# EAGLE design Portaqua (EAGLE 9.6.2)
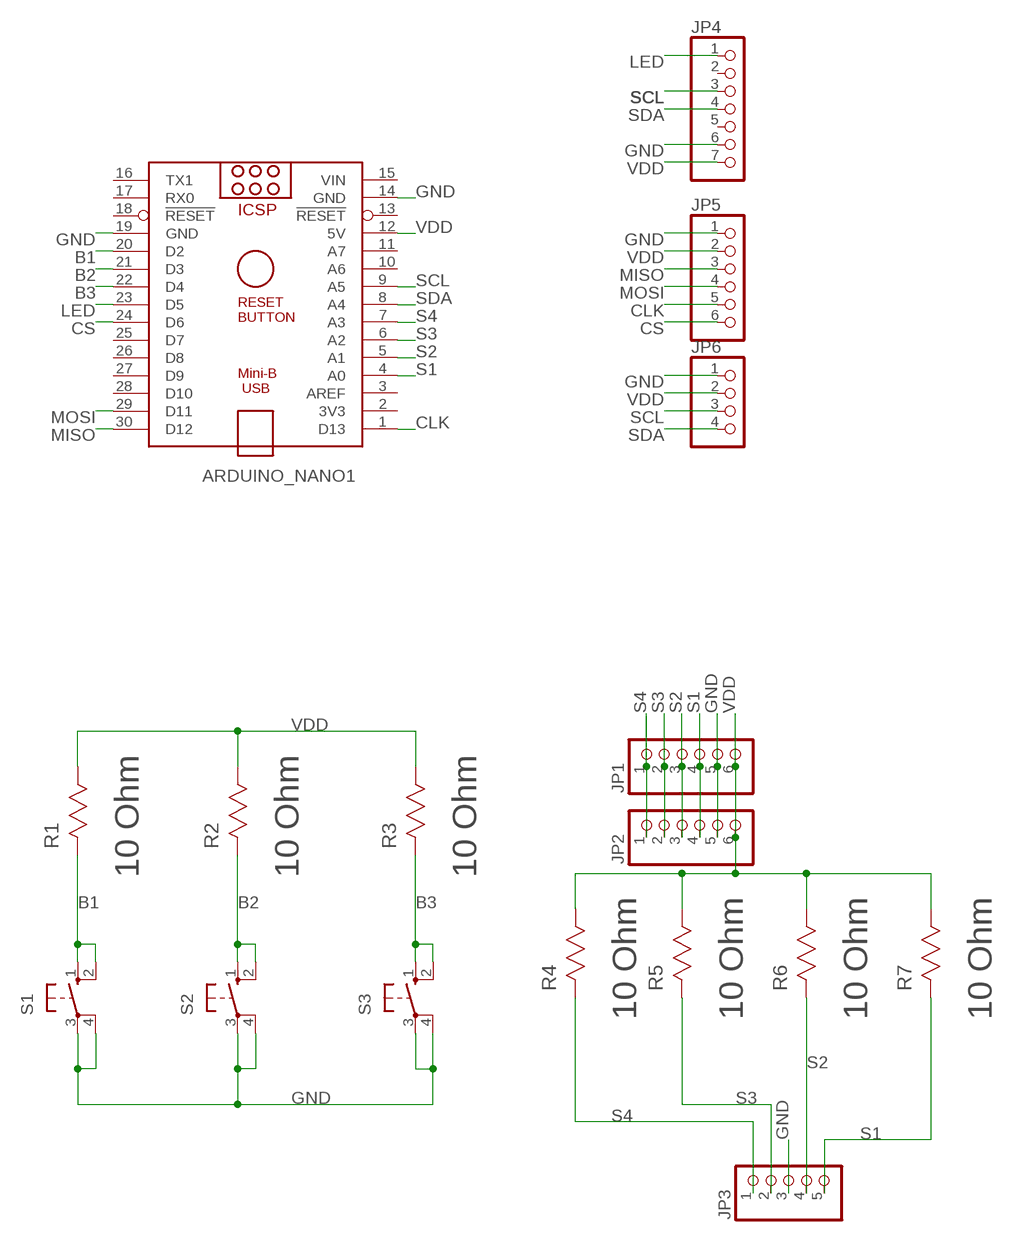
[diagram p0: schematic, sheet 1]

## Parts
ARDUINO_NANO1  ARDUINO_NANO  [ARDUINO_NANO]
JP1  PINHD-1X6  [1X06]
JP2  PINHD-1X6  [1X06]
JP3  PINHD-1X05_2.54-SMD-90°  [1X05SMD/90]
JP4  PINHD-1X7  [1X07]
JP5  PINHD-1X6  [1X06]
JP6  PINHD-1X4  [1X04]
R1  10 Ohm  CRM1206-FX-10R0ELF  [RESC3216X71N]
R2  10 Ohm  CRM1206-FX-10R0ELF  [RESC3216X71N]
R3  10 Ohm  CRM1206-FX-10R0ELF  [RESC3216X71N]
R4  10 Ohm  CRM1206-FX-10R0ELF  [RESC3216X71N]
R5  10 Ohm  CRM1206-FX-10R0ELF  [RESC3216X71N]
R6  10 Ohm  CRM1206-FX-10R0ELF  [RESC3216X71N]
R7  10 Ohm  CRM1206-FX-10R0ELF  [RESC3216X71N]
S1  10-XX  [B3F-10XX]
S2  10-XX  [B3F-10XX]
S3  10-XX  [B3F-10XX]

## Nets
B1: ARDUINO_NANO1.20(D2) R1.2(R2) S1.1(S) S1.2(S1)
B2: ARDUINO_NANO1.21(D3) R2.2(R2) S2.1(S) S2.2(S1)
B3: ARDUINO_NANO1.22(D4) R3.2(R2) S3.1(S) S3.2(S1)
CLK: ARDUINO_NANO1.1(D13) JP5.5
CS: ARDUINO_NANO1.24(D6) JP5.6
GND: ARDUINO_NANO1.14(GND) ARDUINO_NANO1.19(GND) JP1.5 JP2.5 JP3.3 JP4.6 JP5.1 JP6.1 S1.3(P) S1.4(P1) S2.3(P) S2.4(P1) S3.3(P) S3.4(P1)
LED: ARDUINO_NANO1.23(D5) JP4.1
MISO: ARDUINO_NANO1.30(D12) JP5.3
MOSI: ARDUINO_NANO1.29(D11) JP5.4
S1: ARDUINO_NANO1.4(A0) JP1.4 JP2.4 JP3.5 R7.2(R2)
S2: ARDUINO_NANO1.5(A1) JP1.3 JP2.3 JP3.4 R6.2(R2)
S3: ARDUINO_NANO1.6(A2) JP1.2 JP2.2 JP3.2 R5.2(R2)
S4: ARDUINO_NANO1.7(A3) JP1.1 JP2.1 JP3.1 R4.2(R2)
SCL: ARDUINO_NANO1.9(A5) JP4.3 JP6.3
SDA: ARDUINO_NANO1.8(A4) JP4.4 JP6.4
VDD: ARDUINO_NANO1.12(5V) JP1.6 JP2.6 JP4.7 JP5.2 JP6.2 R1.1(R1) R2.1(R1) R3.1(R1) R4.1(R1) R5.1(R1) R6.1(R1) R7.1(R1)
Unconnected: ARDUINO_NANO1.2(3V3) ARDUINO_NANO1.3(AREF) ARDUINO_NANO1.10(A6) ARDUINO_NANO1.11(A7) ARDUINO_NANO1.13(!RESET) ARDUINO_NANO1.16(TX1) ARDUINO_NANO1.17(RX0) ARDUINO_NANO1.18(!RESET) ARDUINO_NANO1.25(D7) ARDUINO_NANO1.26(D8) ARDUINO_NANO1.27(D9) ARDUINO_NANO1.28(D10) JP4.2 JP4.5

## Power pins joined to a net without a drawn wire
VIN: ARDUINO_NANO1.15(VIN)

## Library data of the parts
ARDUINO_NANO1 = ArduinoNanoV30:ARDUINO_NANO: Arduino Nano V3.0 Overview: The Arduino Nano is a small, complete, and breadboard-friendly board based on the ATmega328 (Arduino Nano 3.x) or ATmega168 (Arduino Nano 2.x). It has more or less the same functionality of the Arduino Duemilanove, but in a different package. It lacks only a DC power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
JP1 JP2 JP5 = pinhead:PINHD-1X6: PIN HEADER
JP3 = pinhead-2:PINHD-1X05: PIN HEADER
JP4 = pinhead:PINHD-1X7: PIN HEADER
JP6 = pinhead:PINHD-1X4: PIN HEADER
R1-R7 = Bourns_By_element14_Batch_1:CRM1206-FX-10R0ELF: Resistor 1206; MPN: CRM1206-FX-10R0ELF; OC_FARNELL: 1865248; OC_NEWARK: 17T4257; SUPPLIER: BOURNS; TOLERANCE: ±1 %; WATTAGE: 0.5W
S1-S3 = switch-omron:10-XX: OMRON SWITCH; MPN: B3F-1000; OC_FARNELL: 176432; OC_NEWARK: 36M3542

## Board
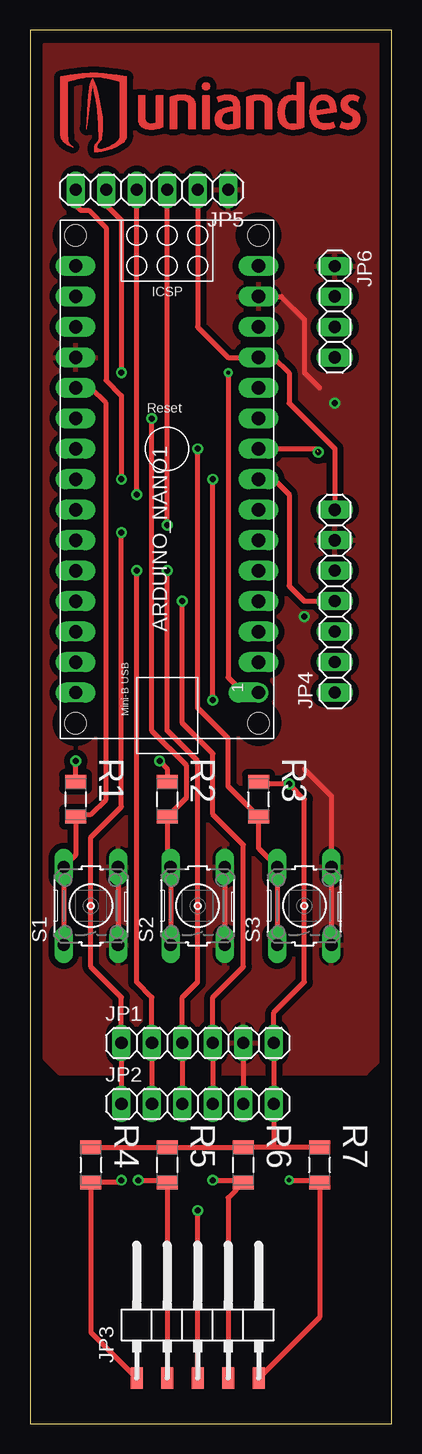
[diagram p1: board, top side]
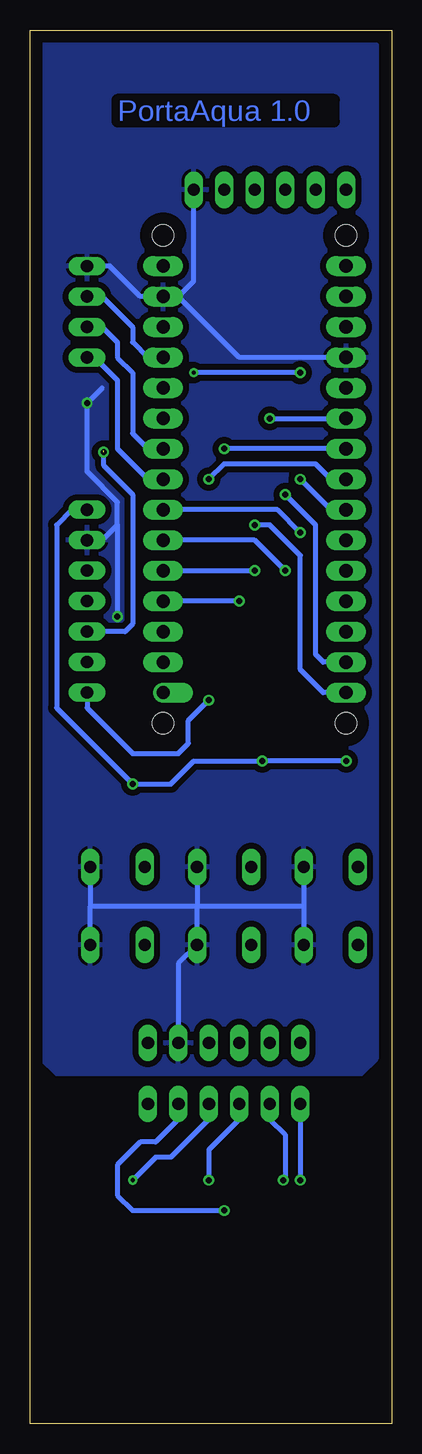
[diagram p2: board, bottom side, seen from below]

Size 30.15 x 116.2 mm. Coordinates in mm from the lower left corner, seen from the top.
Outline: 0,0 30.15,0 30.15,116.2 0,116.2 0,0
Copper layers (1*16): Top 0.035mm / dielectric 1.5mm / Bottom 0.035mm
Design rules "default *": minimum track width 6mil, minimum drill 0.35mm, track to track 20mil, track to pad 20mil, pad to pad 20mil, via to via 20mil, smd to smd 20mil, copper to edge 40mil, drill to drill 6mil, minimum pad ring 10mil, minimum via ring 8mil, stop-mask expansion 4mil, vias tented up to drill 0mil, thermal gap 10mil

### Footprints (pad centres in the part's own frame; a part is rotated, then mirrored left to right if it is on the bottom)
ARDUINO_NANO = drill 1.11 offset: 1 -20.32,-7.62 | drill 1.11 long: 2 -17.78,-7.62; 3 -15.24,-7.62; 4 -12.7,-7.62; 5 -10.16,-7.62; 6 -7.62,-7.62; 7 -5.08,-7.62; 8 -2.54,-7.62; 9 0,-7.62; 10 2.54,-7.62; 11 5.08,-7.62; 12 7.62,-7.62; 13 10.16,-7.62; 14 12.7,-7.62; 15 15.24,-7.62; 16 15.24,7.62; 17 12.7,7.62; 18 10.16,7.62; 19 7.62,7.62; 20 5.08,7.62; 21 2.54,7.62; 22 0,7.62; 23 -2.54,7.62; 24 -5.08,7.62; 25 -7.62,7.62; 26 -10.16,7.62; 27 -12.7,7.62; 28 -15.24,7.62; 29 -17.78,7.62; 30 -20.32,7.62 | hole 1.778: -22.86,-7.62; -22.86,7.62; 17.78,7.62; 17.78,-7.62
1X06 = drill 1.016 long: 1 -6.35,0; 2 -3.81,0; 3 -1.27,0; 4 1.27,0; 5 3.81,0; 6 6.35,0
1X05SMD/90 = smd 1.016 x 1.778: 1 -1.27,-5.08; 2 1.27,-5.08; 3 3.81,-5.08; 4 6.35,-5.08; 5 8.89,-5.08
1X07 = drill 1.016 long: 1 -7.62,0; 2 -5.08,0; 3 -2.54,0; 4 0,0; 5 2.54,0; 6 5.08,0; 7 7.62,0
1X04 = drill 1.016 long: 1 -3.81,0; 2 -1.27,0; 3 1.27,0; 4 3.81,0
RESC3216X71N = smd 1.118 x 1.753: 1 -1.473,0; 2 1.473,0
B3F-10XX = drill 1.016 long: 1 -3.251,2.261; 2 3.251,2.261; 3 -3.251,-2.261; 4 3.251,-2.261

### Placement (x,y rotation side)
ARDUINO_NANO1  11.43,81.28 90 top
JP1  13.97,31.75 0 top
JP2  13.97,26.67 0 top
JP3  10.16,8.89 0 top
JP4  25.4,68.58 90 top
JP5  10.16,102.87 180 top
JP6  25.4,92.71 270 top
R1  3.81,52.07 270 top
R2  11.43,52.07 270 top
R3  19.05,52.07 270 top
R4  5.08,21.59 270 top
R5  11.43,21.59 270 top
R6  17.78,21.59 270 top
R7  24.13,21.59 270 top
S1  5.08,43.18 90 top
S2  13.97,43.18 90 top
S3  22.86,43.18 90 top
U$1  [UNIANDES25MM]  2.54,106.05 0 top

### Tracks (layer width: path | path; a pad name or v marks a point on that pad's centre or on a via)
B1
  Top 0.406: S1.1 S1.2 3.81,47.42 R1.2 4.01,50.8 5.08,50.8 6.35,52.07 6.35,85.09 5.08,86.36 ARDUINO_NANO1.20
B2  (via drill 0.5)
  Top 0.406: S2.1 S2.2 11.43,46.71 R2.2 13.06,52.22 13.06,54.87 10.16,57.76 v10.16,83.82
  Bottom 0.406: v10.16,83.82 ARDUINO_NANO1.21
B3  (via drill 0.5)
  Top 0.406: S3.1 S3.2 19.05,47.98 R3.2 16.51,53.14 16.51,57.15 13.97,59.69 v13.97,81.28
  Bottom 0.406: ARDUINO_NANO1.22 v13.97,81.28
CLK  (via drill 0.35, 0.5)
  Top 0.406: v7.62,87.63 7.62,100.33 6.35,101.6 JP5.5 | ARDUINO_NANO1.1 17.78,60.96 16.51,62.23 v16.51,87.63
  Bottom 0.406: v7.62,87.63 v16.51,87.63
CS  (via drill 0.5)
  Top 0.406: v7.62,78.74 7.62,85.73 6.35,87 6.35,99.7 4.88,101.17 4.24,101.17 3.81,101.6 JP5.6
  Bottom 0.406: v7.62,78.74 5.08,76.2 ARDUINO_NANO1.24
GND  (via drill 0.5)
  Top 0.406: JP1.5 JP2.5 | JP3.3 v13.97,17.78 | 24.13,86.36 22.86,87.63 22.86,92.08 20.95,93.98 ARDUINO_NANO1.14 | 22.86,54.61 25.12,52.35 S3.4 S3.3 | S2.4 S2.3 | S1.4 S1.3
  Bottom 0.406: S1.4 7.34,43.18 | 7.34,43.18 S1.3 | S2.4 16.23,43.18 | 16.23,43.18 S2.3 17.78,38.38 JP1.5 | S3.4 25.12,43.18 | S3.3 25.12,43.18 | 25.12,43.18 16.23,43.18 | 16.23,43.18 7.34,43.18 | v13.97,17.78 21.59,17.78 22.86,19.05 22.86,21.59 20.95,23.5 19.68,23.5 17.78,25.4 JP2.5 | 17.78,93.98 12.7,88.9 ARDUINO_NANO1.19 | 17.78,93.98 ARDUINO_NANO1.14 20.95,93.98 23.5,96.52 JP6.1 | 17.78,93.98 16.51,95.25 JP5.1 | JP4.6 24.13,73.66 22.86,74.93 | 22.86,74.93 22.86,76.84 25.4,79.38 v25.4,85.09 24.13,86.36 | 22.86,74.93 v22.86,67.31
  pour Top: 1.27,114.94 29.21,114.94 29.21,30.48 27.94,29.21 2.54,29.21 1.27,30.48
  pour Bottom: 2.54,29.21 1.27,30.48 1.27,114.94 29.21,114.94 29.21,30.48 27.94,29.21
LED  (via drill 0.5)
  Top 0.406: v15.24,60.33 v15.24,78.74
  Bottom 0.406: JP4.1 25.4,59.69 21.59,55.88 17.78,55.88 16.94,56.72 16.94,58.62 v15.24,60.33 | ARDUINO_NANO1.23 5.08,78.74 6.35,80.01 13.97,80.01 v15.24,78.74
MISO  (via drill 0.5)
  Top 0.406: v11.43,74.93 JP5.3
  Bottom 0.406: v11.43,74.93 10.16,74.93 7.62,72.39 7.62,62.87 5.71,60.96 ARDUINO_NANO1.30
MOSI  (via drill 0.5)
  Top 0.406: v8.89,77.47 JP5.4
  Bottom 0.406: ARDUINO_NANO1.29 5.71,63.5 6.35,64.14 6.35,74.93 v8.89,77.47
S1  (via drill 0.35, 0.5)
  Top 0.406: JP2.4 JP1.4 15.24,35.56 17.78,38.1 17.78,48.26 15.24,50.8 15.24,55.88 12.7,58.42 v12.7,68.58 | v21.59,20.32 23.93,20.32 R7.2 24.13,8.89 JP3.5
  Bottom 0.406: v21.59,20.32 19.68,22.22 18.41,22.22 15.24,25.4 JP2.4 | v12.7,68.58 ARDUINO_NANO1.4
S2  (via drill 0.5)
  Top 0.406: JP2.3 JP1.3 12.7,35.56 13.97,36.83 13.97,55.25 11.43,57.78 v11.43,71.12 | v15.24,20.32 17.58,20.32 R6.2 16.51,18.85 JP3.4
  Bottom 0.406: v15.24,20.32 15.24,22.86 12.7,25.4 JP2.3 | ARDUINO_NANO1.5 v11.43,71.12
S3  (via drill 0.5)
  Top 0.406: JP2.2 JP1.2 10.16,35.56 8.89,36.83 v8.89,71.12 | JP3.2 R5.2 11.23,20.32 v9.03,20.32
  Bottom 0.406: JP2.2 10.16,25.4 8.89,24.13 8.89,20.32 v9.03,20.32 | ARDUINO_NANO1.6 11.43,73.66 v8.89,71.12
S4  (via drill 0.5)
  Top 0.406: JP2.1 JP1.1 7.62,35.56 5.08,38.1 5.08,48.89 7.62,51.44 v7.62,74.3 | v7.62,20.32 7.42,20.12 R4.2 5.08,7.62 JP3.1
  Bottom 0.406: JP2.1 v7.62,20.32 | ARDUINO_NANO1.7 9.53,76.2 v7.62,74.3
SCL  (via drill 0.5)  (1 unrouted)
  Top 0.406: 24,81.14 23.86,81.28 ARDUINO_NANO1.9
  Bottom 0.406: JP6.3 24.13,91.44 22.86,90.17 22.86,88.9 21.59,87.63 21.59,82.55 20.32,81.28 ARDUINO_NANO1.9 | JP4.3 22.23,66.04 21.59,66.67 21.59,77.47 24,79.88 24,81.14 24.02,81.12 v24.02,81.01
SDA
  Top 0.406: ARDUINO_NANO1.8 20.32,78.74 21.59,77.47 21.59,69.85 22.86,68.58 JP4.4
  Bottom 0.406: ARDUINO_NANO1.8 20.32,78.74 21.59,80.01 22.86,81.28 22.86,82.55 22.86,87 24.77,88.9 JP6.4
VDD  (via drill 0.5)
  Top 0.406: R4.1 R5.1 R6.1 20.32,23.06 | R7.1 20.32,23.06 | 20.32,23.06 JP2.6 JP1.6 20.32,34.29 22.86,36.83 22.86,52.07 v21.59,53.34 19.25,53.34 R3.1 | JP5.2 13.97,91.44 16.51,88.9 ARDUINO_NANO1.12 20.32,88.9 21.59,87.63 21.59,85.09 25.4,81.28 JP4.7 | v10.79,55.25 11.43,54.61 R2.1 | R1.1 v3.81,55.25
  Bottom 0.406: JP6.2 24.13,93.98 21.59,91.44 21.59,90.17 20.32,88.9 ARDUINO_NANO1.12 | JP4.7 26.67,76.2 27.94,74.93 27.94,59.69 v21.59,53.34 18.41,53.34 16.51,55.25 v10.79,55.25 v3.81,55.25

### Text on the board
Bottom: PortaAqua 1.0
